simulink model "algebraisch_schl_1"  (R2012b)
settings: Solver=ode45  StartTime=0.0  StopTime=1  RelTol=1e-3
libraries: simulink x1

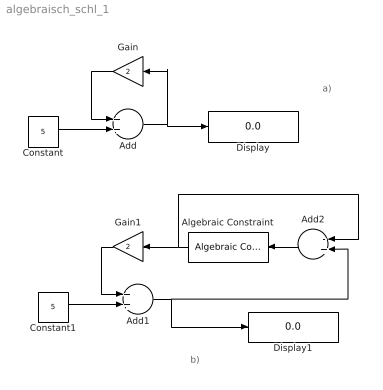
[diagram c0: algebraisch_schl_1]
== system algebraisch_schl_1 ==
  note: b)
  note: a)
  Add : Sum
  Add1 : Sum
  Add2 : Sum  Inputs=-+
  Algebraic Constraint : simulink/Math Operations/Algebraic Constraint  z0=0
  Constant : Constant  Value=5
  Constant1 : Constant  Value=5
  Display : Display
  Display1 : Display
  Gain : Gain  Gain=2
  Gain1 : Gain  Gain=2
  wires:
  Constant/1 -> Add/2
  Gain/1 -> Add/1
  Add/1 -> Gain/1, Display/1
  Constant1/1 -> Add1/2
  Gain1/1 -> Add1/1
  Algebraic Constraint/1 -> Add2/1, Gain1/1
  Add2/1 -> Algebraic Constraint/1
  Add1/1 -> Add2/2, Display1/1
